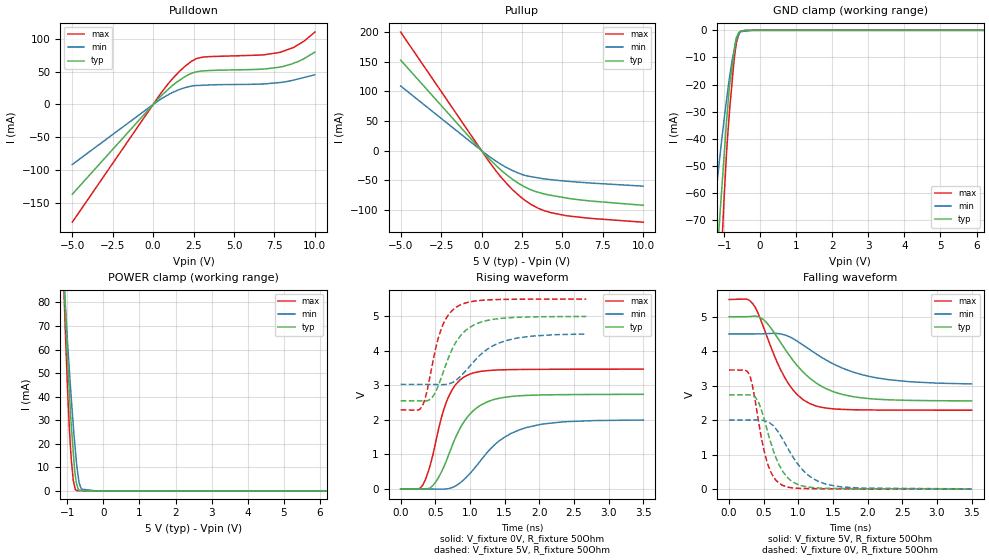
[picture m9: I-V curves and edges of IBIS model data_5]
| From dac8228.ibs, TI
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|   data_5 Model
[Model]   data_5
Model_type   I/O
Polarity   Non-Inverting
Enable   Active-Low
Vinl = 0.8
Vinh = 3.8
Vmeas = 2.5
Vref = 2.5
Cref = 10pF
Rref = 50
|   typ   min   max
|   (nom PVT)   (Fast PVT)   (slow PVT)
|C_comp from frequency method(F=50MHz)
C_comp   8.654e-12   7.287e-12   1.007e-11
|ON state : BUFFER OUTPUT TURNED HIGH
|C_comp   8.654e-12   7.287e-12   1.007e-11
|OFF state: BUFFER IN HIGH IMPEDANCE
|C_comp   8.307e-12   6.941e-12   9.648e-12
|C_comp from L-C Tank method(L=1nH)
|Average
|C_comp   8.186e-12   6.812e-12   9.0955e-12
|ON state : BUFFER OUTPUT TURNED HIGH
|Resonant Frequency(Hz)   1.76e9   1.9e9   1.65e9
|C_comp   8.186e-12   7.024e-12   9.313e-12
|OFF state: BUFFER IN HIGH IMPEDANCE
|Resonant Frequency(Hz)   1.81e9   1.96e9   1.69e9
|C_comp   7.74ee-12   6.6e-12   8.878e-12
| Where nom  PVT is Nominal Process,  5V,  33C
|   Fast PVT is Strong Process,   5.5V,  -40C
|   Slow PVT is Weak Process,   4.5V,  113C
[Voltage Range]   5   4.5   5.5
|Ambient Temperature   25   105   -40
|Junction Temperature
[Temperature Range]   33   113   -40
[Pullup Reference]   5   4.5   5.5
[Pulldown Reference]   0   0   0
[Power Clamp Reference]   5   4.5   5.5
[GND Clamp Reference]   0   0   0
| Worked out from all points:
|   slope of the pulldown table from 0 to 0.75 V, typ, clamps not added: 39.7 ohm
|   slope of the pullup table from 0 to 0.75 V, typ, clamps not added: 35.4 ohm
|   GND clamp passes 1 mA (typ) near -0.60 V on its own axis
|   POWER clamp passes 1 mA (typ) near -0.70 V on its own axis
|   falling waveform, V_fixture 5V, R_fixture 50Ohm: 20-80 % time 621ps typ, 837ps min, 436ps max; typ from 5 V to 2.56 V
|   rising waveform, V_fixture 0V, R_fixture 50Ohm: 20-80 % time 410ps typ, 608ps min, 290ps max; typ from 0 V to 2.74 V
|   rising waveform, V_fixture 5V, R_fixture 50Ohm: 20-80 % time 343ps typ, 492ps min, 244ps max; typ from 2.55 V to 5 V
|   falling waveform, V_fixture 0V, R_fixture 50Ohm: 20-80 % time 281ps typ, 415ps min, 204ps max; typ from 2.74 V to 0.005 V
[Pulldown]
|   Voltage   I(typ)   I(min)   I(max)
-5V       -136.5mA   -91.21mA   -178.9mA
528mV     13.89mA    8.876mA    18.73mA
1.221V    29.43mA    18.44mA    39.85mA
2.007V    42.76mA    25.78mA    58.81mA
2.684V    49.65mA    28.82mA    69.89mA
3.08V     51.01mA    29.23mA    71.98mA
6.6V      53.49mA    31mA       75.06mA
7.854V    56.91mA    33.43mA    79.28mA
8.684V    62.67mA    37.04mA    86.67mA
9.345V    69.89mA    41.09mA    96.42mA
10V       79.54mA    45.11mA    110mA
[GND Clamp]
|   Voltage   I(typ)   I(min)   I(max)
-5V       -981.7mA   -687.3mA   -1.357A
-1.368V   -120.3mA   -78.69mA   -173.2mA
-1.228V   -91.1mA    -60.29mA   -129.3mA
-1.14V    -72.57mA   -49.33mA   -102.3mA
-1.089V   -62.95mA   -43.03mA   -86.87mA
-1.001V   -46.36mA   -32.99mA   -61.99mA
-929.5mV  -33.02mA   -25.32mA   -44.54mA
-855mV    -20.97mA   -17.76mA   -30.72mA
-693mV    -5.221mA   -5.274mA   -7.735mA
-670mV    -2.985mA   -4.048mA   -5.704mA
-544.5mV  -503.3uA   -473.7uA   -353.4uA
10V       0A         0A         0A
[Pullup]
|   Voltage   I(typ)   I(min)   I(max)
-5V       152.3mA    108.7mA    199.5mA
440mV     -12.91mA   -9.14mA    -17.6mA
1.144V    -31.41mA   -22.17mA   -42.77mA
1.672V    -43.23mA   -30.28mA   -59.04mA
2.525V    -58.89mA   -40.38mA   -80.39mA
3.08V     -66.28mA   -43.93mA   -90.92mA
3.547V    -70.52mA   -46.17mA   -97.62mA
4.274V    -75.16mA   -48.89mA   -104.4mA
5.192V    -79.59mA   -51.36mA   -109.4mA
6.84V     -85.12mA   -54.79mA   -114.3mA
10V       -92.12mA   -59.88mA   -120.6mA
[POWER Clamp]
|   Voltage   I(typ)   I(min)   I(max)
-5V       1.399A     1.179A     1.687A
-1.111V   95.69mA    93.54mA    92.87mA
-1.056V   76.86mA    79.04mA    67.78mA
-984.5mV  52.94mA    60.5mA     39.43mA
-907.5mV  31.53mA    42.75mA    16.99mA
-836mV    16.41mA    27.83mA    4.45mA
-795mV    8.276mA    20.19mA    1.601mA
-742.5mV  2.885mA    11.14mA    115.5uA
-679.5mV  421.1uA    3.912mA    105.7uA
-612mV    201.1uA    759.8uA    95.21uA
-202.5mV  26.43nA    5.18nA     31.5uA
10V       0A         0A         0A
[Ramp]
R_load = 50
|   typ   min   max
dV/dt_r   1.64708/4.10832e-10   1.20553/6.18564e-10   2.08166/2.90022e-10
dV/dt_f   1.46775/6.22652e-10   0.882593/8.60065e-10   1.92648/4.35516e-10
[Falling Waveform]
V_fixture = 5V
V_fixture_min = 4.5V
V_fixture_max = 5.5V
R_fixture = 50Ohm
|   Time   V(typ)   V(min)   V(max)
0s        5V         4.5V       5.5V
260ps     5.002V     4.5V       5.507V
344ps     5.013V     4.5V       5.373V
534ps     4.846V     4.508V     4.499V
805ps     4.069V     4.471V     3.234V
977ps     3.599V     4.298V     2.756V
1.165ns   3.217V     4.046V     2.481V
1.537ns   2.805V     3.599V     2.324V
2.049ns   2.621V     3.259V     2.297V
3.5ns     2.561V     3.052V     2.29V
[Rising Waveform]
V_fixture = 0V
V_fixture_min = 0V
V_fixture_max = 0V
R_fixture = 50Ohm
|   Time   V(typ)   V(min)   V(max)
0s        3.535nV    4.449nV    3.247nV
322ps     -3.667mV   327.3uV    125.7mV
416ps     24.1mV     -84.58uV   618.4mV
496ps     174.3mV    -1.408mV   1.27V
669ps     864.2mV    4.598mV    2.565V
794ps     1.499V     90.72mV    3.022V
951ps     2.052V     346.4mV    3.284V
1.399ns   2.617V     1.357V     3.446V
1.814ns   2.71V      1.778V     3.462V
3.5ns     2.741V     1.997V     3.47V
[Rising Waveform]
V_fixture = 5V
V_fixture_min = 4.5V
V_fixture_max = 5.5V
R_fixture = 50Ohm
|   Time   V(typ)   V(min)   V(max)
0s        2.554V     3.029V     2.289V
309ps     2.549V     3.029V     2.389V
365ps     2.547V     3.029V     2.711V
466ps     2.681V     3.027V     3.697V
586ps     3.224V     3.021V     4.638V
682ps     3.758V     3.037V     5.021V
808ps     4.285V     3.164V     5.27V
1.041ns   4.732V     3.656V     5.433V
1.413ns   4.933V     4.221V     5.487V
2.677ns   4.995V     4.487V     5.499V
[Falling Waveform]
V_fixture = 0V
V_fixture_min = 0V
V_fixture_max = 0V
R_fixture = 50Ohm
|   Time   V(typ)   V(min)   V(max)
0s        2.736V     2.005V     3.456V
291ps     2.732V     2.006V     3.328V
352ps     2.702V     2.007V     2.858V
422ps     2.53V      2.005V     2.012V
548ps     1.733V     1.963V     796.4mV
649ps     1.064V     1.815V     334mV
775ps     516.1mV    1.447V     111.1mV
1.073ns   87.47mV    536.7mV    20.42mV
1.421ns   25.43mV    134.1mV    11.63mV
3.5ns     5.324mV    9.92mV     962.2uV
